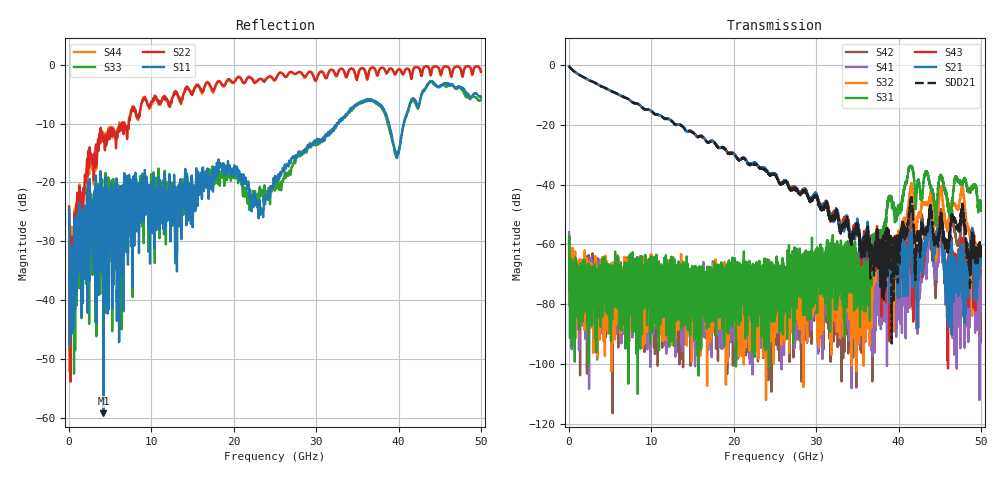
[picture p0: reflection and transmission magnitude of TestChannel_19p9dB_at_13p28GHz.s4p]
# GHz S MA R 50
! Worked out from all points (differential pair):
!   5000 points, 10 MHz to 50 GHz, reference 50 ohm
!   strongest paths, dB at 10 MHz, 12.51 GHz, 25.01 GHz, 37.51 GHz, 50 GHz:
!     S21: -0.5, -18.8, -36.3, -57.9, -63.9
!     S43: -0.4, -18.9, -36.8, -61.2, -61.9
!     S31: -63.5, -71.7, -80.4, -57.9, -47.9
!     S32: -57.9, -71.9, -85.1, -60.7, -64.5
!     S41: -55.9, -73.4, -72.6, -71.8, -74.9
!     S42: -57.0, -73.0, -78.0, -62.2, -68.3
!   taken as a pair (ports 1,3 in; 2,4 out), SDD21 dB: -0.4, -18.9, -36.8, -64.0, -61.3
!   lowest |S11| = -59.3 dB at 4.17 GHz (marker M1), VSWR 1.00, Z = 50.1 + j0.0108 ohm
!   |S11| at or under -10 dB: start of sweep to 32.53 GHz; 32.54234 GHz to 32.58446 GHz (42.11 MHz wide, 0.129 % of centre); 38.83 GHz to 40.63 GHz (1.792 GHz wide, 4.51 % of centre)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
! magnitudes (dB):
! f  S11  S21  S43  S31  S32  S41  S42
! 10 MHz  -24.6  -0.5  -0.4  -63.5  -57.9  -55.9  -57.0
! 4.17 GHz  -59.3  -7.4  -7.4  -69.8  -68.8  -72.2  -71.9
! 35.55 GHz  -6.2  -60.2  -63.0  -63.0  -72.5  -77.3  -81.7
! 41.52 GHz  -6.1  -59.7  -63.7  -34.0  -40.1  -57.9  -49.0
! 45.75 GHz  -3.2  -76.7  -71.6  -43.0  -53.2  -70.8  -72.9
! 47.75 GHz  -4.0  -77.8  -65.6  -39.9  -40.7  -62.8  -47.4
! 50 GHz  -5.5  -63.9  -61.9  -47.9  -64.5  -74.9  -68.3
